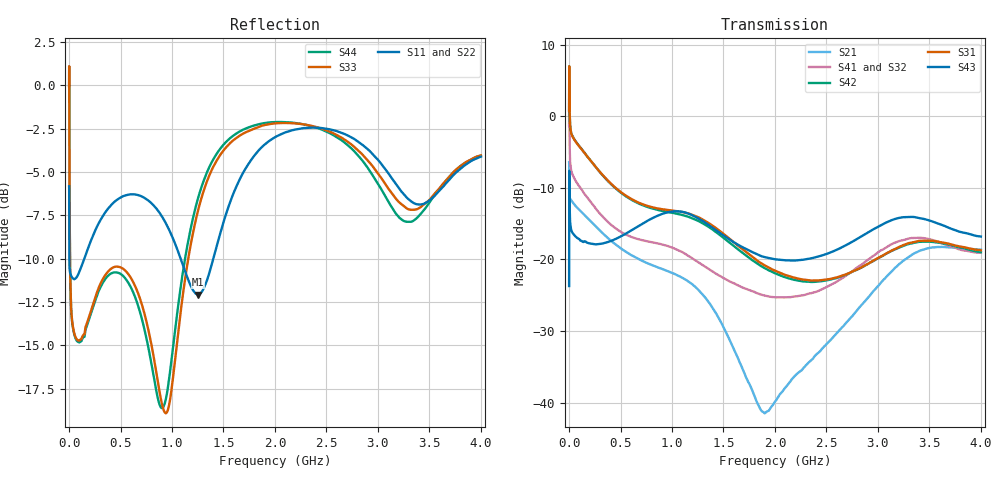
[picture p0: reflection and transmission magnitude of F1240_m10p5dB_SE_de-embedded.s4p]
! Integrated Device Technology
! Corporate Headquarters
! 6024 Silver Creek Valley Road
! San Jose, CA 95138  USA
! Phone:  1-408-284-8200
! Toll Free:  1-800-223-1366
! Webpage:  http://www.idt.com/
! Timing and RF Division
! 515 Groton Road, Suite 102
! Westford, MA 01886-6024
! Device:  F1240
! Description: Dual Intermediate Frequency Digital Variable Gain Amplifier
! Frequency:  10.0 -  500.00 MHz
! Package:  5x5 mm QFN Plastic Package: 32 pin
! Ports:  8 RF, 20 DC
!  Pin  1  = GA3 / Data  Pin 17  = RF OUT_B+
!  Pin  2  = GA4 / CLK  Pin 18  = RF OUT_B-
!  Pin  3  = GA5  Pin 19  = STBY_B
!  Pin  4  = VMODE  Pin 20  = Ground
!  Pin  5  = No Connect  Pin 21  = Ground
!  Pin  6  = GB5  Pin 22  = STB_A
!  Pin  7  = GB4  Pin 23  = RF OUT_A-  = Port 4
!  Pin  8  = GB3  Pin 24  = RF OUT_A+  = Port 3
!  Pin  9  = GB2  Pin 25  = GA0
!  Pin 10  = GB1  Pin 26  = ISET_A
!  Pin 11  = RF IN_B+  Pin 27  = VCC
!  Pin 12  = RF IN_B-  Pin 28  = Ground
!  Pin 13  = Ground  Pin 29  = RF IN_A-  = Port 2
!  Pin 14  = VCC  Pin 30  = RF IN_A+  = Port 1
!  Pin 15  = ISET_B  Pin 31  = GA1
!  Pin 16  = GB0  Pin 32  = GA2 / CSb
! Gain  = +19.5 dB
! State  = 1
! Voltage  = +5.00 V
! Current  = 85.292 mA (one channel only)
! Temperture  =  +25 C
! Test Date  =  2017-10-18
! Board  =  EB4031
! Data:  The device was measured on a custom evaluation board which has
!  individual transmission lines to the RF pins.  Data was collected
!  using a calibrated network analyzer.  The evaluation board was
!  de-embedded using Automatic Fixture Removal.
!  The reference plane is the edge of the package pin.
!  Only Channel A was measured.
!  This data is in single-ended operation.  If your needs are balanced
!  or differential S-parameters then this file needs to be used a
!  linear simulator.
! File Date:  2017-11-10  MJV
! Note:
!  Integrated Device Technology supplies this data as a sample of measured
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# Hz S dB R 100
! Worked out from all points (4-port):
!   410 points, 500 kHz to 4 GHz, reference 100 ohm
!   strongest paths, dB at 500 kHz, 930 MHz, 1.96 GHz, 2.98 GHz, 4 GHz:
!     S43: -23.7, -13.5, -19.9, -15.6, -16.8
!     S31: 0.8, -13.0, -21.3, -20.0, -18.7
!     S42: 0.8, -13.3, -21.6, -20.0, -19.0
!     S41: -1.3, -18.0, -25.2, -19.3, -19.0
!     S32: -1.2, -18.2, -25.0, -19.4, -19.3
!     S21: -6.4, -21.5, -40.7, -24.1, -18.6
!   lowest |S11| = -12.1 dB at 1.25 GHz (marker M1), VSWR 1.66, Z = 60.9 - j9.06 ohm
!   |S11| at or under -10 dB: 3.076 MHz to 148.4 MHz (145.3 MHz wide, 192 % of centre); 1.084 GHz to 1.401 GHz (317.2 MHz wide, 25.5 % of centre)
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500000  -5.82 -5.6  -6.42 -5.8  -31.95 76.4  -33.93 75.7
        -6.43 -5.8  -5.82 -5.6  -33.92 74.5  -31.94 77.5
        0.80 -112.2  -1.25 -113.9  -0.04 -0.4  -23.70 -38.4
        -1.26 -112.8  0.79 -111.0  -23.71 -38.5  -0.05 1.9
3500000  -10.22 -17.1  -11.03 -15.9  -25.76 2.4  -29.78 -11.1
         -11.03 -15.9  -10.22 -17.3  -29.74 -11.2  -25.76 2.6
         2.78 154.1  -1.23 140.7  -4.12 -84.9  -10.05 174.3
         -1.26 140.9  2.79 154.3  -10.07 174.3  -4.17 -84.9
3.7e8  -7.18 -124.1  -16.92 -98.8  -30.78 -79.7  -37.24 -78.7
       -16.92 -98.7  -7.10 -124.8  -37.34 -77.0  -30.96 -79.6
       -8.89 58.6  -14.74 24.3  -10.80 -163.7  -17.66 48.1
       -14.66 23.5  -8.95 57.3  -17.60 47.7  -11.04 -164.5
1.25e9  -12.06 -163.7  -24.26 96.1  -30.18 122.2  -35.50 151.6
        -24.16 96.1  -11.92 -163.3  -35.27 155.0  -31.52 125.9
        -14.08 -134.8  -20.25 151.0  -7.28 -117.6  -14.39 172.1
        -20.35 143.6  -14.59 -136.0  -14.23 172.2  -6.57 -120.2
1.9e9  -3.42 -166.3  -41.06 46.7  -33.48 6.0  -36.20 27.3
       -41.47 44.7  -3.32 -166.9  -36.56 32.8  -34.87 12.7
       -20.82 91.1  -24.80 25.1  -2.29 -173.8  -19.87 54.1
       -25.04 18.3  -21.20 93.7  -19.68 55.0  -2.18 -176.8
2.84e9  -3.39 111.9  -26.38 -7.4  -29.81 -133.4  -32.20 -120.1
        -26.39 -7.3  -3.22 112.5  -32.67 -107.8  -31.07 -124.7
        -21.12 -50.2  -20.88 -127.0  -3.93 105.0  -17.45 -79.7
        -20.73 -138.0  -21.12 -46.8  -16.77 -77.5  -4.27 98.3
4e9  -4.11 -127.6  -18.62 124.6  -27.23 -18.3  -28.28 -3.5
     -18.62 124.7  -3.88 -126.2  -28.89 9.5  -28.93 -7.6
     -18.72 59.3  -19.28 -34.2  -4.05 -132.9  -18.18 61.3
     -19.05 -48.1  -18.99 65.5  -16.80 55.3  -4.05 -142.8
